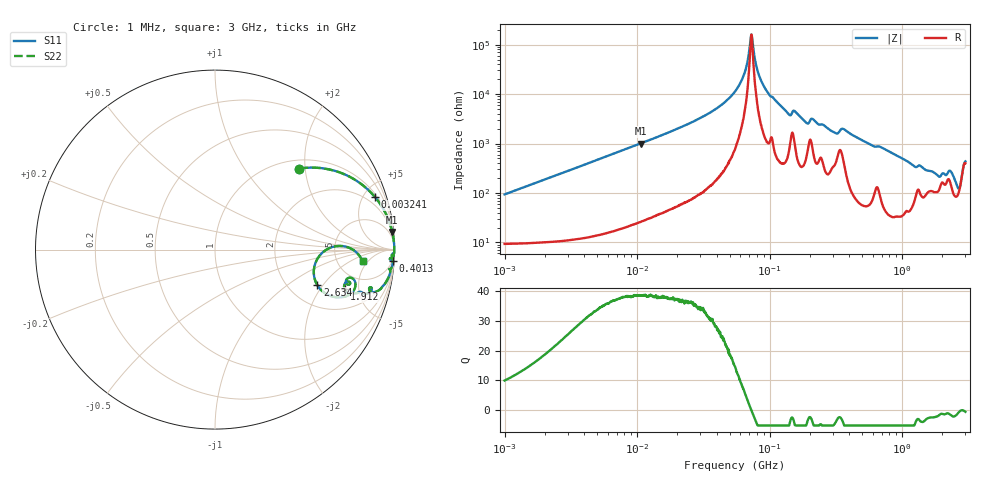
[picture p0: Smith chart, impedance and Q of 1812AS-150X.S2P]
!s-Parameter Generated by FASTRON Sdn. Bhd.
!FASTRON P/N : 1812AS-150X
!Keysight Technologies,E4991B,MY54100416,A.01.15
!Date created: Mon Oct 16 09:44:27 2023
!Version  : Rev00 Mon Oct 16 09:44:27 2023
!Data & Calibration Information:
!Freq	S11	S21	S12	S22
!PortZ  Port1:50+j0  Port2:50+j0
!When reading, reference impedance value at option line is always used.
! Remarks : This data is being provided solely for informational purposes.
# Hz S dB R 50
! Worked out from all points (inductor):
!   1601 points, 1 MHz to 3 GHz, reference 50 ohm
!   read as one part in series: L = 14.8 uH near 1.041 MHz
!   highest Q = 38.4 at 10.61 MHz (marker M1), where L = 15 uH
!   self-resonance near 72.85 MHz
!   S11 on the Smith chart (normalised r, x): 1 MHz: 1.19, +1.87; 3.241 MHz: 1.23, +6.04; 401.3 MHz: 4, -32; 1.912 GHz: 3.42, -3.51; 2.634 GHz: 2.84, -1.76; 3 GHz: 8.98, -3.52
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1000000  -3.71 43.8  -3.15 -40.5  -3.15 -40.5  -3.71 43.8
3241173  -0.55 18.1  -10.15 -69.8  -10.15 -69.8  -0.55 18.1
3804036  -0.41 15.6  -11.41 -72.5  -11.41 -72.5  -0.41 15.6
1.061086e7  -0.07 5.7  -20.07 -82.8  -20.07 -82.8  -0.07 5.7
1.447069e7  -0.04 4.1  -22.86 -84.4  -22.86 -84.4  -0.04 4.1
3.491183e7  -0.01 1.4  -32.28 -86.8  -32.28 -86.8  -0.01 1.4
5.477226e7  -0.01 0.5  -41.03 -85.6  -41.03 -85.6  -0.01 0.5
6.428402e7  -0.01 0.2  -48.12 -80.9  -48.12 -80.9  -0.01 0.2
7.321605e7  -0.01 -0.0  -63.93 12.3  -63.93 12.3  -0.01 -0.0
8.29729e7  -0.01 -0.2  -47.69 80.6  -47.69 80.6  -0.01 -0.2
9.836149e7  -0.01 -0.6  -40.05 83.7  -40.05 83.7  -0.01 -0.6
1.396205e8  -0.04 -1.4  -31.86 78.5  -31.86 78.5  -0.04 -1.4
1.904091e8  -0.08 -2.1  -28.36 75.2  -28.36 75.2  -0.08 -2.1
2.083556e8  -0.08 -1.7  -30.16 71.2  -30.16 71.2  -0.08 -1.7
3.10929e8  -0.13 -3.3  -24.52 73.7  -24.52 73.7  -0.13 -3.3
4.013235e8  -0.06 -3.5  -24.22 81.9  -24.22 81.9  -0.06 -3.5
7.925923e8  -0.15 -8.1  -17.00 78.9  -17.00 78.9  -0.15 -8.1
1.912199e9  -2.44 -17.0  -9.01 38.5  -9.01 38.5  -2.44 -17.0
2.289646e9  -1.93 -13.0  -10.94 39.4  -10.94 39.4  -1.93 -13.0
2.634014e9  -4.40 -19.1  -6.49 24.6  -6.49 24.6  -4.40 -19.1
2.811057e9  -3.43 1.6  -9.70 -3.3  -9.70 -3.3  -3.43 1.6
3e9  -1.68 -4.4  -14.48 19.4  -14.48 19.4  -1.68 -4.4
